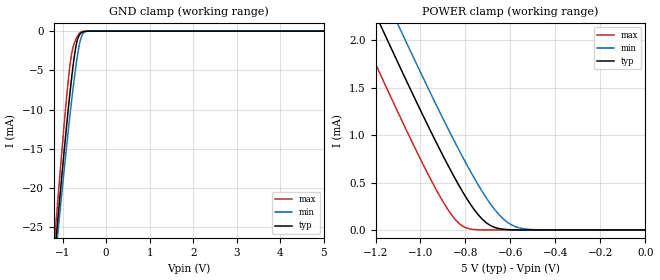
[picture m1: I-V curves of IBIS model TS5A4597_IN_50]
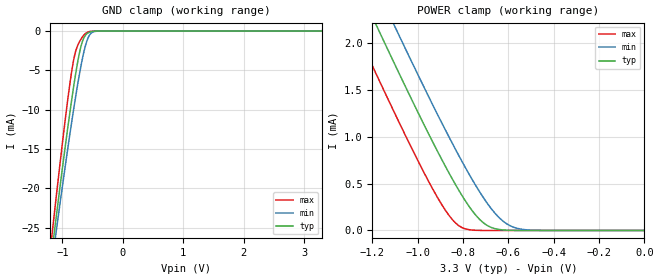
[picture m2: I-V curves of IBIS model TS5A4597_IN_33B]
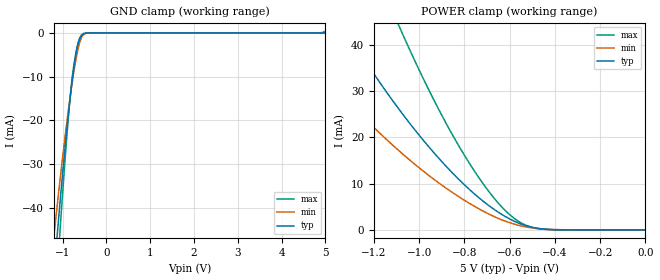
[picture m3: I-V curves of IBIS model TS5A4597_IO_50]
| TEXAS INSTRUMENTS INCORPORATED
| Standard Linear and Logic Group
| IBIS Model of TS5A4597
| SINGLE-CHANNEL 8-OHM SPST ANALOG SWITCH
| This file contains package information for the following:
|  SOT 5-pin (DBV) package as [Component] TS5A4597_DBV
|  SOT 5-pin (DCK) package as [Component] TS5A4597_DCK
| This device can be POWERed at the following Vccs:
|  5 volt Vcc
|  3.3 volt Vcc
| This file provides unique models under the [Model Selector] for each Vcc.
| For operation at a specific Vcc, select the appropriate model after each
| [Model Selector] keyword.
[IBIS Ver]   3.2
[Comment char]  |_char
[File Name]   ts5a4597.ibs
[File Rev]   1.1 | x_die
[Date]   January 26, 2005
[Source]   Data created from TI-SPICE simulations at TI-SLL.
[Notes]   The following is an IBIS list for the TS5A4597.
   Please contact sllibis@ti.com with questions and
   comments concerning SLL IBIS models.
   - FILE REV HISTORY
   - 1.1 Release IBIS file on 02/02/05
   - Non-monotonic data due to FET characteristics.
   - NCH & PCH MOSFETS, so [Series Mosfet] model can have rising
   or falling currents
[Disclaimer] Property of Texas Instruments Incorporated.  Unauthorized
   reproduction and/or distribution is strictly prohibited.
   This product is protected under copyright law.
   Created  2005, (C) Copyright  2005, Texas Instruments
   Incorporated, All Rights Reserved
   UNLESS THERE IS A SIGNED, WRITTEN AGREEMENT TO THE
   CONTRARY, TEXAS INSTRUMENTS (TI) IS PROVIDING THE IBIS
   MODELS  AND WITHOUT ANY WARRANTY, EXPRESSED OR
   IMPLIED.  TI assumes no liability for:
   1) the accuracy of the IBIS models provided to your
   company;
   2) the proper functioning of these IBIS Models in your
   design or for any resulting applications; or
   3) infringement of patents, copyrights or intellectual
   property rights resulting from your use of these IBIS
   models.
   TI provides IBIS Models as a service to our customers.
   You and your company shall not distribute, sell or give
   these models to anyone else without prior written
   permission from TI.
   TI reserves the right to make changes to our products or
   to discontinue any semiconductor product or service
   without notice, and advises our customers to obtain the
   latest version of relevant information to verify, before
   placing orders, that the information being relied on is
   current.
   Please be aware that your receipt and use of the IBIS
   information provided shall serve as acceptance of these
   terms and conditions.  If you do not accept these terms,
   you should return or destroy the IBIS models and any
   other accompanying information immediately.
| Component TS5A4597_DBV 5-pin SOT
[Component]   TS5A4597_DBV
[Manufacturer]   Texas Instruments, Inc.
[Package]
|   typ   min   max
R_pkg   2.500e-02   2.100e-02   2.900e-02
L_pkg   1.529e-09   1.312e-09   1.906e-09
C_pkg   1.560e-13   1.100e-13   2.400e-13
[Pin]   signal_name   model_name   R_pin   L_pin   C_pin
1   IN   TS5A4597_IN   2.100e-02   1.511e-09   1.440e-13
2   COM   TS5A4597_IO   2.300e-02   1.312e-09   1.380e-13
3   GND   GND   2.900e-02   1.906e-09   2.400e-13
4   NC   TS5A4597_IO   2.600e-02   1.541e-09   1.500e-13
5   VPLUS   POWER   2.500e-02   1.374e-09   1.100e-13
| Component TS5A4597_DCK 5-pin SOT
[Component]   TS5A4597_DCK
[Manufacturer]   Texas Instruments, Inc.
[Package]
|   typ   min   max
R_pkg   2.000e-02   1.700e-02   2.500e-02
L_pkg   9.980e-10   8.810e-10   1.069e-09
C_pkg   1.460e-13   1.180e-13   2.050e-13
[Pin]   signal_name   model_name   R_pin   L_pin   C_pin
1   IN   TS5A4597_IN   1.900e-02   1.069e-09   1.620e-13
2   COM   TS5A4597_IO   1.800e-02   8.810e-10   1.210e-13
3   GND   GND   1.700e-02   1.031e-09   2.050e-13
4   NC   TS5A4597_IO   2.000e-02   9.600e-10   1.240e-13
5   VPLUS   POWER   2.500e-02   1.049e-09   1.180e-13
[Series Switch Groups]
| Function Group States
On  1 /   | COM->NC IN LOW
Off 1 /   | IN HIGH
[Series Pin Mapping]   pin_2   model_name   function_table_group
2   4   TS5A4597_IO_50_S   1
| 2   4   TS5A4597_IO_33B_S   1
| Model TS5A4597_IN
[Model Selector]   TS5A4597_IN
TS5A4597_IN_50   5 volt Vcc
TS5A4597_IN_33B   3.3 volt Vcc
| Model TS5A4597_IO
[Model Selector]   TS5A4597_IO
TS5A4597_IO_50   5 volt Vcc_
TS5A4597_IO_33B   3.3 volt Vcc
| Model TS5A4597_IO_S
[Model Selector]   TS5A4597_IO_S
TS5A4597_IO_50_S   5 volt Vcc_S
TS5A4597_IO_33B_S   3.3 volt Vcc_S
[Model]   TS5A4597_IO_50_S
Model_type  Series_switch
| variable   typ   min   max
C_comp   0   0   0
[Temperature Range]   40   100   -40
| Ambient temperature   25   85   -40
[Voltage range]   5   4.5   5.5
[On]
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[Off]
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[Model]   TS5A4597_IO_33B_S
Model_type  Series_switch
| variable   typ   min   max
C_comp   0   0   0
[Temperature Range]   40   100   -40
| Ambient temperature   25   85   -40
[Voltage range]   3.3   2.7   3.6
[On]
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[Off]
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| Models and submodels in the file (6): TS5A4597_IN_50 (Input), TS5A4597_IN_33B (Input), TS5A4597_IO_50_S (Series_switch), TS5A4597_IO_50 (Terminator), TS5A4597_IO_33B_S (Series_switch), TS5A4597_IO_33B (Terminator)
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[Model]   TS5A4597_IN_50
Model_type  Input
Vinl=0.8
Vinh=2.0
| variable   typ   min   max
C_comp   2.20pF   1.77pF   3.00pF
[Temperature Range]   40   100   -40
| Ambient temperature   25   85   -40
[Voltage range]   5   4.5   5.5
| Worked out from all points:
|   GND clamp passes 1 mA (typ) near -0.65 V on its own axis
|   POWER clamp passes 1 mA (typ) near -0.95 V on its own axis
[GND Clamp]
| TS5A4597_IN_50
|   Voltage   I(typ)   I(min)   I(max)
-5V       -298.4mA   -277.9mA   -323.1mA
-1.19V    -29.14mA   -30.52mA   -27.21mA
-1.155V   -26.94mA   -28.51mA   -24.77mA
-1.12V    -24.77mA   -26.51mA   -22.35mA
-1.085V   -22.61mA   -24.52mA   -19.96mA
-925mV    -13.12mA   -15.71mA   -9.575mA
-820mV    -7.411mA   -10.29mA   -3.964mA
-770mV    -4.979mA   -7.865mA   -2.332mA
-685mV    -1.759mA   -4.156mA   -944.2uA
-565mV    -197.5uA   -717.2uA   -100.3uA
-405mV    -3.947uA   -11.29uA   -534.4nA
5V        90.92pA    3.943uA    64.59pA
[POWER Clamp]
| TS5A4597_IN_50
|   Voltage   I(typ)   I(min)   I(max)
-5V       22.89mA    23.25mA    22.43mA
-1.275V   2.666mA    3.07mA     2.144mA
-1.165V   2.096mA    2.501mA    1.573mA
-1.095V   1.738mA    2.143mA    1.216mA
-1.075V   1.637mA    2.041mA    1.115mA
-930mV    924.4uA    1.32mA     424.7uA
-840mV    516.5uA    894.5uA    96.42uA
-795mV    334.5uA    692.7uA    21.02uA
-725mV    113.3uA    404.3uA    835.8nA
-620mV    5.152uA    92.62uA    5.201nA
-500mV    69.32nA    3.943uA    103.9pA
-84.45fV  90.92pA    203.6pA    76.32pA
[Model]   TS5A4597_IN_33B
Model_type  Input
Vinl=0.8
Vinh=2.0
| variable   typ   min   max
C_comp   2.29pF   1.91pF   2.95pF
[Temperature Range]   40   100   -40
| Ambient temperature   25   85   -40
[Voltage range]   3.3   2.7   3.6
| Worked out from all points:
|   GND clamp passes 1 mA (typ) near -0.65 V on its own axis
|   POWER clamp passes 1 mA (typ) near -0.95 V on its own axis
[GND Clamp]
| TS5A4597_IN_33B
|   Voltage   I(typ)   I(min)   I(max)
-3.3V     -174.9mA   -164.2mA   -188.3mA
-1.175V   -28.2mA    -29.66mA   -26.16mA
-1.145V   -26.32mA   -27.93mA   -24.07mA
-1.09V    -22.92mA   -24.8mA    -20.3mA
-935mV    -13.69mA   -16.25mA   -10.18mA
-825mV    -7.668mA   -10.54mA   -4.177mA
-770mV    -4.979mA   -7.865mA   -2.332mA
-700mV    -2.205mA   -4.76mA    -1.131mA
-590mV    -322.8uA   -1.174mA   -183.5uA
-520mV    -74.82uA   -249uA     -28.68uA
-385mV    -2.236uA   -6.525uA   -242.7nA
3.3V      59.09pA    60.28uA    42.64pA
[POWER Clamp]
| TS5A4597_IN_33B
|   Voltage   I(typ)   I(min)   I(max)
-3.3V     13.59mA    13.97mA    13.11mA
-1.275V   2.666mA    3.07mA     2.144mA
-1.185V   2.199mA    2.604mA    1.676mA
-1.105V   1.789mA    2.194mA    1.266mA
-1.07V    1.612mA    2.016mA    1.09mA
-940mV    971.9uA    1.369mA    468.7uA
-845mV    537.9uA    917.5uA    109.5uA
-795mV    334.5uA    692.7uA    21.02uA
-725mV    113.3uA    404.3uA    835.7nA
-625mV    6.134uA    102.3uA    6.579nA
-510mV    99.45nA    5.302uA    85.13pA
-48.03fV  59.09pA    144.7pA    49.79pA
[Model]   TS5A4597_IO_50
Model_type  Terminator
| variable   typ   min   max
C_comp   4.61pF   3.90pF   5.61pF
| C_tri-state   4.61pF   3.90pF   5.61pF
[Temperature Range]   40   100   -40
| Ambient temperature   25   85   -40
[Voltage range]   5   4.5   5.5
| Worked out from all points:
|   GND clamp passes 1 mA (typ) near -0.59 V on its own axis
|   POWER clamp passes 1 mA (typ) near -0.53 V on its own axis
[GND Clamp]
| TS5A4597_IO_50
|   Voltage   I(typ)   I(min)   I(max)
-5V       -653mA     -543.3mA   -770.4mA
-1.2V     -55.59mA   -46.82mA   -66.96mA
-1.16V    -50.72mA   -43mA      -60.69mA
-1.12V    -45.94mA   -39.26mA   -54.53mA
-1.06V    -38.98mA   -33.8mA    -45.53mA
-890mV    -20.82mA   -19.46mA   -22.07mA
-785mV    -11.22mA   -11.7mA    -10.65mA
-730mV    -7.021mA   -8.121mA   -6.573mA
-665mV    -3.3mA     -4.529mA   -3.057mA
-600mV    -1.244mA   -1.916mA   -978.5uA
-530mV    -323.2uA   -492uA     -171uA
5V        394.2pA    428.6uA    63.06pA
[POWER Clamp]
| TS5A4597_IO_50
|   Voltage   I(typ)   I(min)   I(max)
-5V       515.5mA    385.8mA    722.5mA
-1.6V     66.56mA    44.15mA    110.1mA
-1.565V   63.39mA    41.99mA    105.1mA
-1.32V    42.72mA    28.11mA    71.78mA
-1.09V    26.13mA    17.14mA    44.16mA
-1.065V   24.51mA    16.07mA    41.42mA
-910mV    15.31mA    10.05mA    25.7mA
-790mV    9.295mA    6.103mA    15.34mA
-690mV    5.185mA    3.389mA    8.173mA
-580mV    1.9mA      1.264mA    2.515mA
-440mV    168.8uA    146.2uA    110.6uA
-84.45fV  394.2pA    1.79nA     77.08pA
